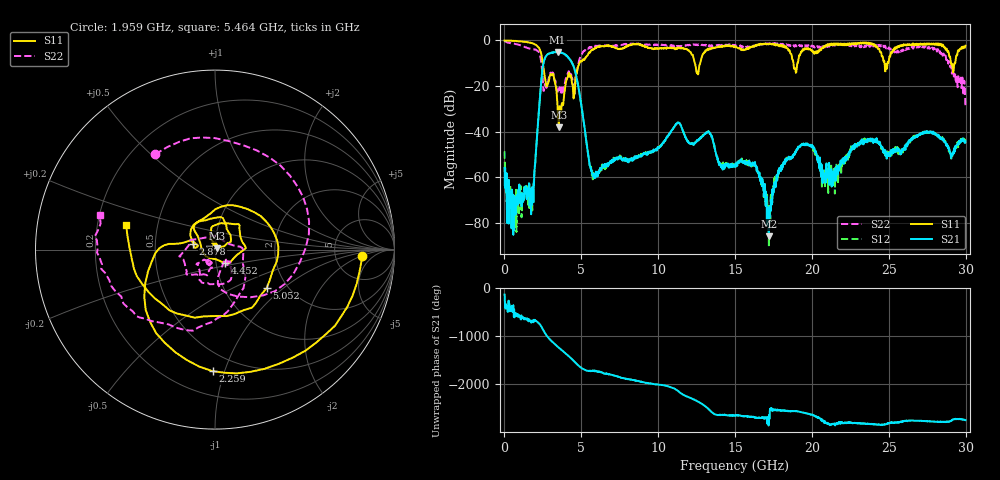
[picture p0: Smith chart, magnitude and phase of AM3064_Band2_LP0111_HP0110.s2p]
# Hz S DB R 50.0
!freq dBS11 angS11 dBS21 angS21 dBS12 angS12 dBS22 angS22
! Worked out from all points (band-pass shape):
!   1600 points, 10 MHz to 29.98 GHz, reference 50 ohm
!   highest |S21| = -5.03 dB at 3.459 GHz (marker M1); lowest = -85.9 dB at 17.2 GHz (marker M2)
!   |S21| within 3 dB of the highest: 2.622 GHz to 4.205 GHz (1.583 GHz wide, 46.4 % of centre)
!   lowest |S11| = -38.0 dB at 3.534 GHz (marker M3), VSWR 1.03, Z = 51.1 + j0.651 ohm
!   |S11| at or under -10 dB: 2.498 GHz to 4.865 GHz (2.367 GHz wide, 64.3 % of centre); 12.38 GHz to 12.73 GHz (343 MHz wide, 2.73 % of centre); 29.04 GHz to 29.32 GHz (271.6 MHz wide, 0.931 % of centre)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
!   |S22| runs from -29.2 to -0.2 dB; largest |S21 - S12| = 0.017
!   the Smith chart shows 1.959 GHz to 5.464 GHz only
!   S11 on the Smith chart (normalised r, x): 1.959 GHz: 9.70, -2.24; 2.259 GHz: 0.36, -0.91; 2.878 GHz: 0.78, +0.05; 4.452 GHz: 1.10, -0.17; 5.052 GHz: 1.57, -0.78; 5.464 GHz: 0.33, +0.12
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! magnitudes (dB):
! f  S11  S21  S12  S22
! 10 MHz  0.0  -56.0  -48.7  -0.2
! 591.1 MHz  -0.2  -67.9  -71.6  -1.4
! 1.959 GHz  -1.7  -56.6  -57.7  -4.1
! 2.259 GHz  -3.4  -29.2  -29.1  -5.5
! 2.878 GHz  -18.1  -5.8  -5.8  -16.8
! 3.459 GHz  -29.6  -5.0  -5.2  -22.6
! 3.534 GHz  -38.0  -5.1  -5.1  -22.4
! 4.452 GHz  -20.6  -10.7  -10.7  -18.8
! 5.015 GHz  -9.3  -29.1  -29.2  -6.3
! 5.052 GHz  -8.9  -30.7  -30.7  -5.8
! 5.464 GHz  -5.8  -51.0  -50.8  -3.5
! 10 GHz  -3.6  -47.2  -46.9  -2.0
! 11.31 GHz  -3.1  -36.1  -36.2  -2.6
! 15 GHz  -2.6  -54.9  -54.5  -2.1
! 16.3 GHz  -2.1  -53.3  -54.5  -2.3
! 17.2 GHz  -1.5  -85.9  -90.2  -1.7
! 18.23 GHz  -3.1  -54.2  -54.3  -1.6
! 19.99 GHz  -4.3  -46.6  -46.9  -2.3
! 21.43 GHz  -2.0  -57.9  -56.8  -1.8
! 25 GHz  -9.0  -50.6  -48.9  -3.1
! 28.31 GHz  -2.0  -42.4  -42.4  -4.7
! 29.98 GHz  -2.4  -44.3  -44.6  -29.2
